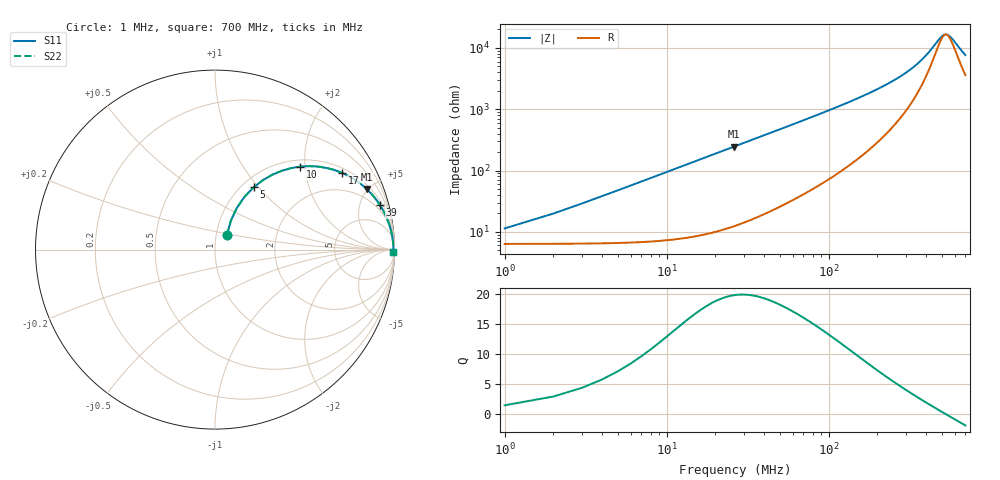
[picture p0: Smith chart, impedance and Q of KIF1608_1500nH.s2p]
# MHz S RI R 50
!Freq ReS11 ImS11 ReS21 ImS21 ReS12 ImS12 ReS22 ImS22
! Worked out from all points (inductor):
!   700 points, 1 MHz to 700 MHz, reference 50 ohm
!   read as one part in series: L = 1.5 uH near 4 MHz
!   highest Q = 19.9 at 26 MHz (marker M1), where L = 1.49 uH
!   self-resonance near 530.6 MHz
!   S11 on the Smith chart (normalised r, x): 1 MHz: 1.13, +0.19; 5 MHz: 1.13, +0.94; 10 MHz: 1.15, +1.88; 17 MHz: 1.18, +3.20; 39 MHz: 1.38, +7.31; 700 MHz: open
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1  0.067 0.0826  0.933 -0.0826  0.933 -0.0826  0.067 0.0826
3  0.1221 0.2329  0.8779 -0.2329  0.8779 -0.2329  0.1221 0.2329
5  0.2148 0.3467  0.7852 -0.3467  0.7852 -0.3467  0.2148 0.3467
7  0.3217 0.4184  0.6783 -0.4184  0.6783 -0.4184  0.3217 0.4184
10  0.4731 0.4621  0.5269 -0.4621  0.5269 -0.4621  0.4731 0.4621
13  0.5942 0.4598  0.4058 -0.4598  0.4058 -0.4598  0.5942 0.4598
17  0.7087 0.4271  0.2913 -0.4271  0.2913 -0.4271  0.7087 0.4271
21  0.7841 0.3861  0.2159 -0.3861  0.2159 -0.3861  0.7841 0.3861
26  0.8445 0.3381  0.1555 -0.3381  0.1555 -0.3381  0.8445 0.3381
39  0.9196 0.2474  0.0804 -0.2474  0.0804 -0.2474  0.9196 0.2474
54  0.953 0.1856  0.047 -0.1856  0.047 -0.1856  0.953 0.1856
72  0.9702 0.1414  0.0298 -0.1414  0.0298 -0.1414  0.9702 0.1414
118  0.9853 0.0855  0.0147 -0.0855  0.0147 -0.0855  0.9853 0.0855
167  0.9901 0.0577  0.00993 -0.0577  0.00993 -0.0577  0.9901 0.0577
234  0.9924 0.037  0.00757 -0.037  0.00757 -0.037  0.9924 0.037
351  0.9937 0.0173  0.00629 -0.0173  0.00629 -0.0173  0.9937 0.0173
467  0.994 0.0052  0.006 -0.0052  0.006 -0.0052  0.994 0.0052
499  0.994 0.00249  0.00599 -0.00249  0.00599 -0.00249  0.994 0.00249
525  0.994 0.000428  0.00599 -0.000428  0.00599 -0.000428  0.994 0.000428
551  0.994 -0.00154  0.00601 0.00154  0.00601 0.00154  0.994 -0.00154
584  0.994 -0.00391  0.00604 0.00391  0.00604 0.00391  0.994 -0.00391
700  0.9938 -0.0114  0.00624 0.0114  0.00624 0.0114  0.9938 -0.0114
